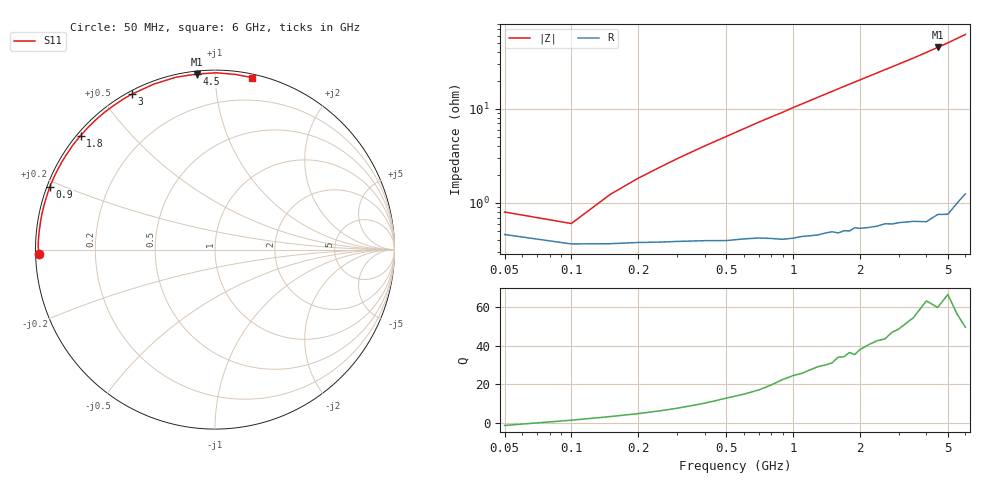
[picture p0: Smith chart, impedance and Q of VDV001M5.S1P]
! Infineon Technologies  Discrete & RF Semiconductors
! BBY 55-03
! Si Tuning Diode in SOD323
! VR =
! S-Parameters:  June  1999
# GHz  S  MA  R  50
!  f  S11
! GHz  MAG  ANG
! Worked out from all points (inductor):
!   34 points, 50 MHz to 6 GHz, reference 50 ohm
!   read as one part to ground: L = 1.42 nH near 150 MHz
!   highest Q = 63.2 at 4.5 GHz (marker M1), where L = 1.6 nH
!   S11 on the Smith chart (normalised r, x): 50 MHz: 0.01, -0.01; 900 MHz: 0.01, +0.18; 1.8 GHz: 0.01, +0.37; 3 GHz: 0.01, +0.60; 4.5 GHz: 0.02, +0.90; 6 GHz: 0.02, +1.24
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0.05  0.9817 -178.5
0.1  0.9855 178.9
0.15  0.9854 177.3
0.2  0.9849 175.9
0.3  0.9846 173.3
0.4  0.9843 170.8
0.5  0.9844 168.4
0.7  0.9835 163.6
0.8  0.9838 161.3
0.9  0.9842 159.1
1  0.9839 156.7
1.2  0.9833 152.3
1.3  0.983 150.1
1.6  0.9828 143.8
1.8  0.9824 139.7
1.9  0.9812 137.8
2  0.9818 135.8
2.2  0.9819 132.0
2.4  0.9818 128.4
2.6  0.9813 124.8
2.8  0.982 121.4
3  0.982 118.1
3.5  0.983 110.3
4  0.9847 102.8
4.5  0.9835 95.8
5  0.9851 89.5
5.5  0.9826 83.3
6  0.9805 77.8
